(* Logix 5000 AddOnInstructionDefinition export GracoCore_DecodeDateTime; software revision 32.04; part 2 of 4 *)

ADD_ON_INSTRUCTION GracoPd2kDual_ReadJobInfo   (* revision 1.0 *)
// Help:
// Reads data from a job record.
// If indexNum is out of range, an error will be raised.
// State Codes:
// * 0000 (IDLE) - Idle
// * 1000 (BUSY) - Busy
// * 2000 (DONE) - Done
// * 4000 (ABORT) - Command overwritten by another process
// * 8000 (ERROR) - Index number out of range
// * 8001 (ERROR) - Timeout waiting for DCS registers
// * 8002 (ERROR) - Command unsuccessful
// * 8003 (ERROR) - Unhandled internal error
VAR_INPUT
   i_execute : BOOL; {visible}   // Execute command
   i_indexNum : DINT; {visible}   // Index number
END_VAR
VAR_IN_OUT
   io_userID : STRING9; {required}   // User ID
   io_moduleStatus : DINT[62]; {required}   // Data from device to PLC
   io_moduleCmds : DINT[30]; {required}   // Data from PLC to device
   io_dateTime : GracoCore_TypeDateTime; {required}   // Alarm/event datetime
END_VAR
VAR_OUTPUT
   o_mixUnitNum : DINT; {access Read Only, visible}   // Mix unit number
   o_jobNum : DINT; {access Read Only, visible}   // Job number
   o_recipeNum : DINT; {access Read Only, visible}   // Recipe number
   o_abVol : DINT; {access Read Only, visible}   // Material A+B used volume (cc)
   o_busy : BOOL; {access Read Only, visible}   // Busy flag
   o_done : BOOL; {access Read Only, visible}   // Done flag
   o_aborted : BOOL; {access Read Only, visible}   // Aborted flag
   o_error : BOOL; {access Read Only, visible}   // Error flag
   o_state : DINT; {access Read Only, visible}   // Command state
END_VAR
VAR
   sendDCSInst : GracoPd2kDual_SendDCS; {access None}   // SendDCS instruction
   decodeDateTime : GracoCore_DecodeDateTime; {access None}   // DecodeDateTime instruction
   decodeUserID : GracoCore_DecodeUserID; {access None}   // DecodeUserID instruction
END_VAR

ROUTINE Logic   (* ladder *)
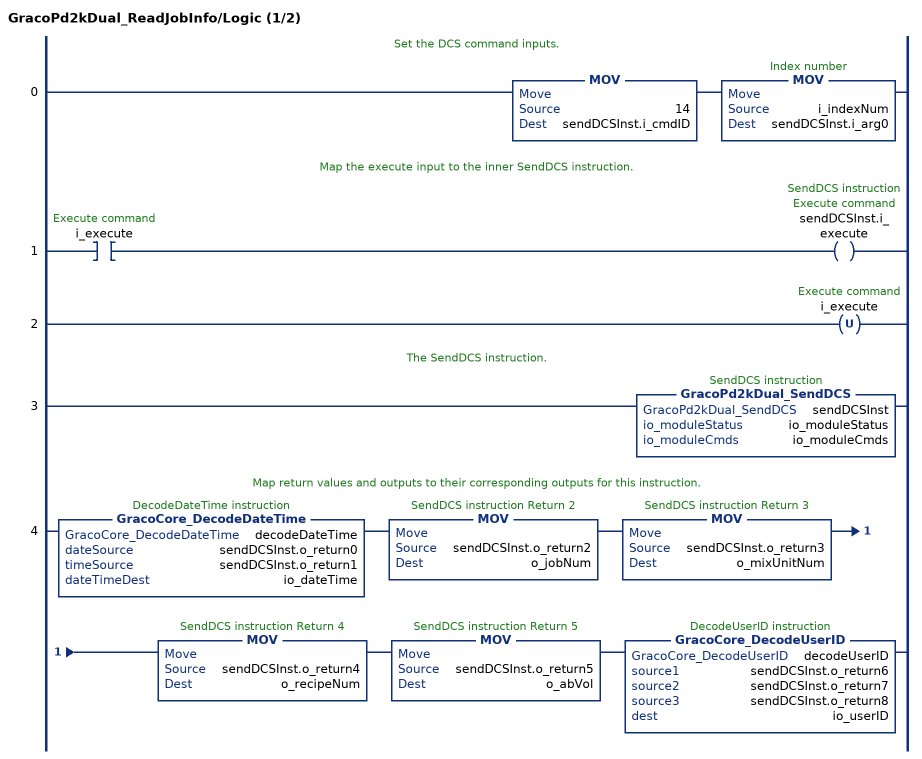
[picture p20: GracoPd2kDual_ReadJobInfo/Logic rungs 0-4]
   // Set the DCS command inputs.
   0: MOV(14,sendDCSInst.i_cmdID)MOV(i_indexNum,sendDCSInst.i_arg0);
   // Map the execute input to the inner SendDCS instruction.
   1: XIC(i_execute)OTE(sendDCSInst.i_execute);
   2: OTU(i_execute);
   // The SendDCS instruction.
   3: GracoPd2kDual_SendDCS(sendDCSInst,io_moduleStatus,io_moduleCmds);
   // Map return values and outputs to their corresponding outputs for this instruction.
   4: GracoCore_DecodeDateTime(decodeDateTime,sendDCSInst.o_return0,sendDCSInst.o_return1,io_dateTime)MOV(sendDCSInst.o_return2,o_jobNum)MOV(sendDCSInst.o_return3,o_mixUnitNum)MOV(sendDCSInst.o_return4,o_recipeNum)MOV(sendDCSInst.o_return5,o_abVol)GracoCore_DecodeUserID(decodeUserID,sendDCSInst.o_return6,sendDCSInst.o_return7,sendDCSInst.o_return8,io_userID);
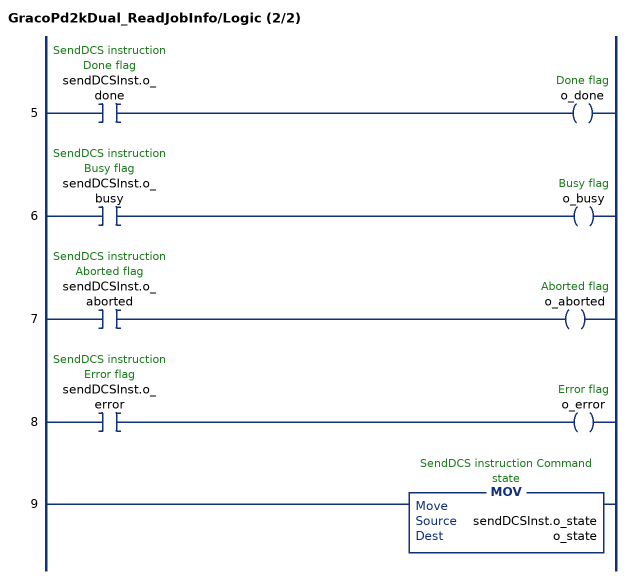
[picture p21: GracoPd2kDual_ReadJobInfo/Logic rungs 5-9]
   5: XIC(sendDCSInst.o_done)OTE(o_done);
   6: XIC(sendDCSInst.o_busy)OTE(o_busy);
   7: XIC(sendDCSInst.o_aborted)OTE(o_aborted);
   8: XIC(sendDCSInst.o_error)OTE(o_error);
   9: MOV(sendDCSInst.o_state,o_state);
END_ROUTINE
END_ADD_ON_INSTRUCTION

ADD_ON_INSTRUCTION GracoPd2kDual_ReadUserID   (* revision 1.0 *)
// Help:
// Returns the current user ID for the system.
// The returned value is a string of up to 9 characters, not including a null terminator.
// State Codes:
// * 0000 (IDLE) - Idle
// * 1000 (BUSY) - Busy
// * 2000 (DONE) - Done
// * 4000 (ABORT) - Command overwritten by another process
// * 8000 (ERROR) - Mix unit number out of range
// * 8001 (ERROR) - Timeout waiting for DCS registers
// * 8002 (ERROR) - Command unsuccessful
// * 8003 (ERROR) - Unhandled internal error
VAR_INPUT
   i_execute : BOOL; {visible}   // Execute command
   i_mixUnitNum : DINT; {visible}   // Mix unit number
END_VAR
VAR_IN_OUT
   io_userID : STRING9; {required}   // User ID
END_VAR
VAR_OUTPUT
   o_busy : BOOL; {access Read Only, visible}   // Busy flag
   o_done : BOOL; {access Read Only, visible}   // Done flag
   o_aborted : BOOL; {access Read Only, visible}   // Aborted flag
   o_error : BOOL; {access Read Only, visible}   // Error flag
   o_state : DINT; {access Read Only, visible}   // Command state
END_VAR
VAR_IN_OUT
   io_moduleStatus : DINT[62]; {required}   // Data from device to PLC
   io_moduleCmds : DINT[30]; {required}   // Data from PLC to device
END_VAR
VAR
   sendDCSInst : GracoPd2kDual_SendDCS; {access None}   // SendDCS instruction
   decodeUserID : GracoCore_DecodeUserID; {access None}   // DecodeUserID instruction
END_VAR

ROUTINE Logic   (* ladder *)
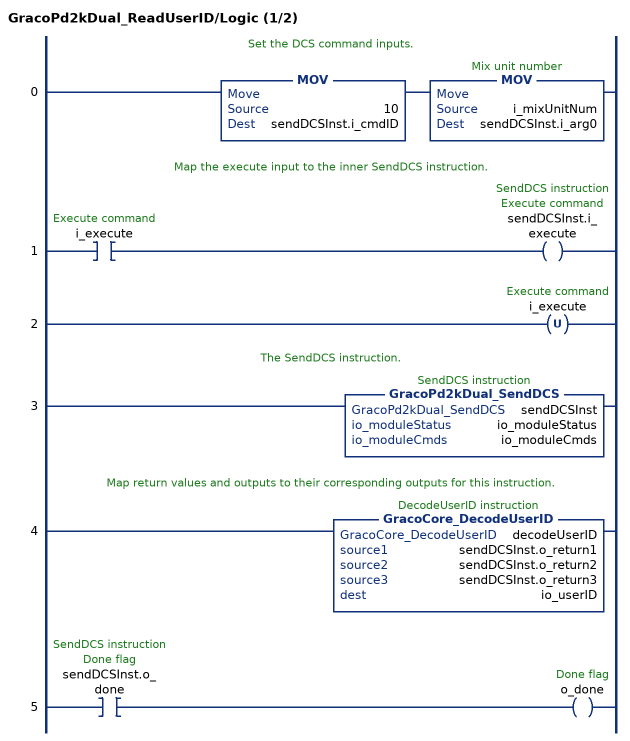
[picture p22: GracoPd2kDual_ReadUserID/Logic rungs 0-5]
   // Set the DCS command inputs.
   0: MOV(10,sendDCSInst.i_cmdID)MOV(i_mixUnitNum,sendDCSInst.i_arg0);
   // Map the execute input to the inner SendDCS instruction.
   1: XIC(i_execute)OTE(sendDCSInst.i_execute);
   2: OTU(i_execute);
   // The SendDCS instruction.
   3: GracoPd2kDual_SendDCS(sendDCSInst,io_moduleStatus,io_moduleCmds);
   // Map return values and outputs to their corresponding outputs for this instruction.
   4: GracoCore_DecodeUserID(decodeUserID,sendDCSInst.o_return1,sendDCSInst.o_return2,sendDCSInst.o_return3,io_userID);
   5: XIC(sendDCSInst.o_done)OTE(o_done);
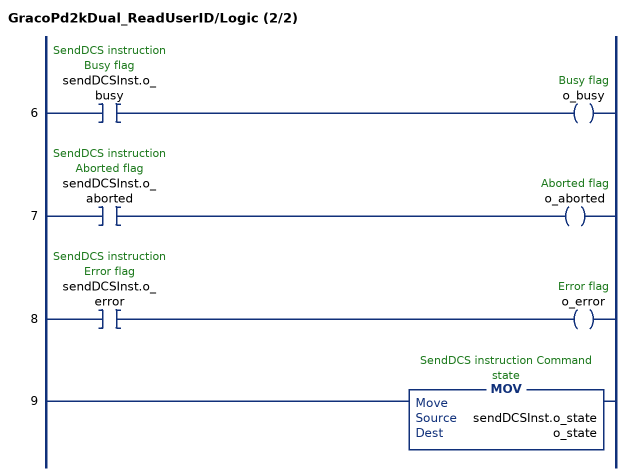
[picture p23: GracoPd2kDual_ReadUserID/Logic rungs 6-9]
   6: XIC(sendDCSInst.o_busy)OTE(o_busy);
   7: XIC(sendDCSInst.o_aborted)OTE(o_aborted);
   8: XIC(sendDCSInst.o_error)OTE(o_error);
   9: MOV(sendDCSInst.o_state,o_state);
END_ROUTINE
END_ADD_ON_INSTRUCTION

ADD_ON_INSTRUCTION GracoCore_EncodeUserID   (* revision 1.0 *)
// Help:
// Parses a user ID String (max 9 characters) into a series of ASCII values stored in DINTs. These can then be written to a Graco CGM.
VAR_IN_OUT
   source : STRING9; {required}
   dest1 : DINT; {required}
   dest2 : DINT; {required}
   dest3 : DINT; {required}
END_VAR
VAR
   buffer : DINT; {access None}
END_VAR

ROUTINE Logic   (* ladder *)
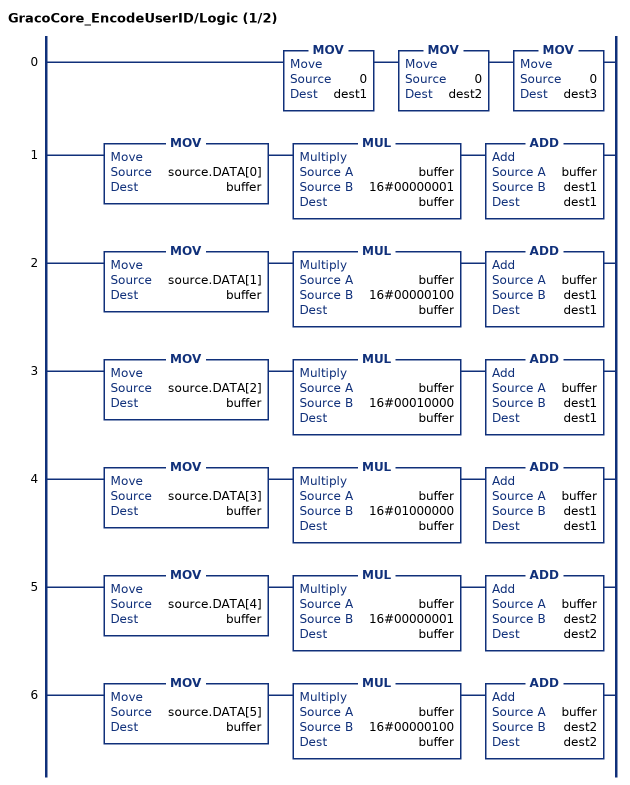
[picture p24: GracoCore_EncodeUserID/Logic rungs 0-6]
   0: MOV(0,dest1)MOV(0,dest2)MOV(0,dest3);
   1: MOV(source.DATA[0],buffer)MUL(buffer,16#00000001,buffer)ADD(buffer,dest1,dest1);
   2: MOV(source.DATA[1],buffer)MUL(buffer,16#00000100,buffer)ADD(buffer,dest1,dest1);
   3: MOV(source.DATA[2],buffer)MUL(buffer,16#00010000,buffer)ADD(buffer,dest1,dest1);
   4: MOV(source.DATA[3],buffer)MUL(buffer,16#01000000,buffer)ADD(buffer,dest1,dest1);
   5: MOV(source.DATA[4],buffer)MUL(buffer,16#00000001,buffer)ADD(buffer,dest2,dest2);
   6: MOV(source.DATA[5],buffer)MUL(buffer,16#00000100,buffer)ADD(buffer,dest2,dest2);
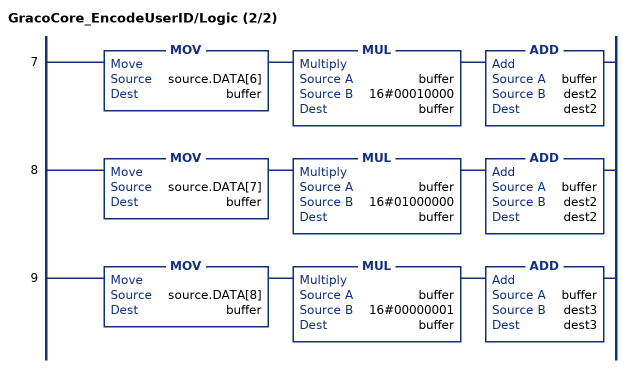
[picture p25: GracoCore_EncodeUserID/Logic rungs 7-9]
   7: MOV(source.DATA[6],buffer)MUL(buffer,16#00010000,buffer)ADD(buffer,dest2,dest2);
   8: MOV(source.DATA[7],buffer)MUL(buffer,16#01000000,buffer)ADD(buffer,dest2,dest2);
   9: MOV(source.DATA[8],buffer)MUL(buffer,16#00000001,buffer)ADD(buffer,dest3,dest3);
END_ROUTINE
END_ADD_ON_INSTRUCTION

ADD_ON_INSTRUCTION GracoPd2kDual_WriteUserID   (* revision 1.0 *)
// Help:
// Sets the current user ID for the system.
// The user ID can be up to 9 characters in length. The value sent to the PD2K will include a null terminator for a total of 10 characters. Only ASCII characters are supported.
// State Codes:
// * 0000 (IDLE) - Idle
// * 1000 (BUSY) - Busy
// * 2000 (DONE) - Done
// * 4000 (ABORT) - Command overwritten by another process
// * 8000 (ERROR) - Mix unit number out of range
// * 8001 (ERROR) - Timeout waiting for DCS registers
// * 8002 (ERROR) - Command unsuccessful
// * 8003 (ERROR) - Unhandled internal error
VAR_INPUT
   i_execute : BOOL; {visible}   // Execute command
END_VAR
VAR_IN_OUT
   io_userID : STRING9; {required}   // User ID
END_VAR
VAR_OUTPUT
   o_busy : BOOL; {access Read Only, visible}   // Busy flag
   o_done : BOOL; {access Read Only, visible}   // Done flag
   o_aborted : BOOL; {access Read Only, visible}   // Aborted flag
   o_error : BOOL; {access Read Only, visible}   // Error flag
   o_state : DINT; {access Read Only, visible}   // Command state
END_VAR
VAR_IN_OUT
   io_moduleStatus : DINT[62]; {required}   // Data from device to PLC
   io_moduleCmds : DINT[30]; {required}   // Data from PLC to device
END_VAR
VAR_INPUT
   i_mixUnitNum : DINT; {visible}   // Mix unit number
END_VAR
VAR
   sendDCSInst : GracoPd2kDual_SendDCS; {access None}   // SendDCS instruction
   encodeUserID : GracoCore_EncodeUserID; {access None}   // EncodeUserID instruction
END_VAR

ROUTINE Logic   (* ladder *)
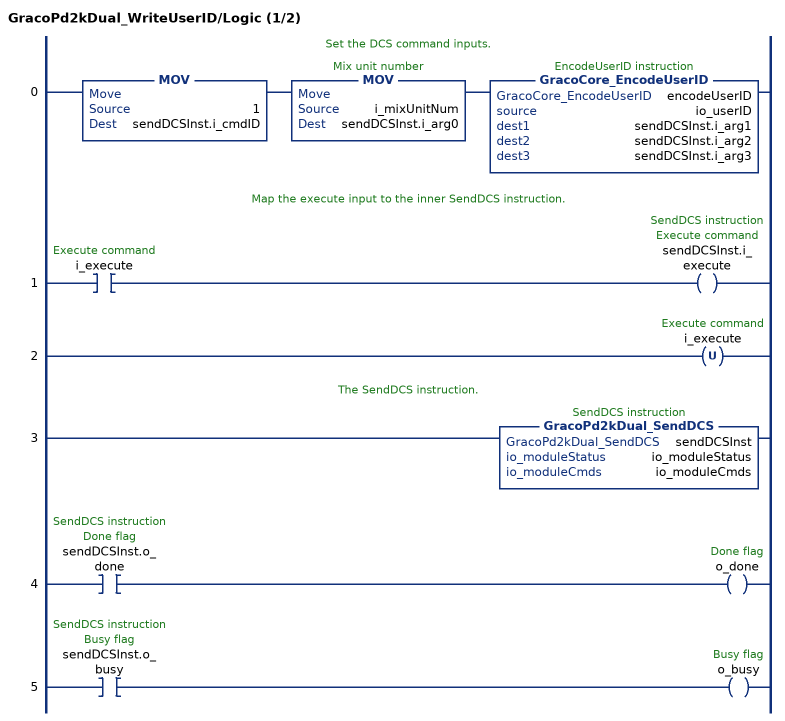
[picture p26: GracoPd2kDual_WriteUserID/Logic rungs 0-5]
   // Set the DCS command inputs.
   0: MOV(1,sendDCSInst.i_cmdID)MOV(i_mixUnitNum,sendDCSInst.i_arg0)GracoCore_EncodeUserID(encodeUserID,io_userID,sendDCSInst.i_arg1,sendDCSInst.i_arg2,sendDCSInst.i_arg3);
   // Map the execute input to the inner SendDCS instruction.
   1: XIC(i_execute)OTE(sendDCSInst.i_execute);
   2: OTU(i_execute);
   // The SendDCS instruction.
   3: GracoPd2kDual_SendDCS(sendDCSInst,io_moduleStatus,io_moduleCmds);
   4: XIC(sendDCSInst.o_done)OTE(o_done);
   5: XIC(sendDCSInst.o_busy)OTE(o_busy);
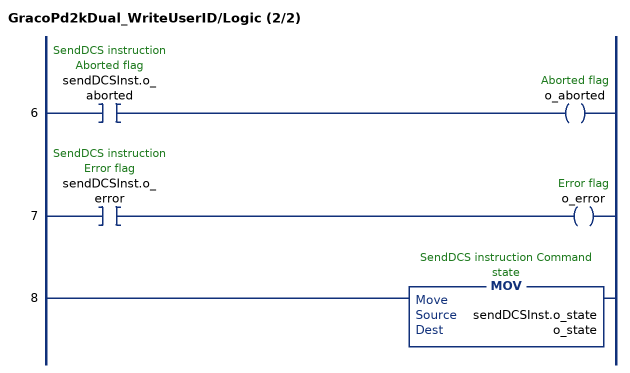
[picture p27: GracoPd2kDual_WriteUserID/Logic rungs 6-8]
   6: XIC(sendDCSInst.o_aborted)OTE(o_aborted);
   7: XIC(sendDCSInst.o_error)OTE(o_error);
   8: MOV(sendDCSInst.o_state,o_state);
END_ROUTINE
END_ADD_ON_INSTRUCTION

ADD_ON_INSTRUCTION GracoCore_Step   (* revision 1.0 *)
// Help:
// An implementation of the step pattern, useful for sequences in ladder logic.
VAR_INPUT
   doneTrigger : BOOL; {access None, visible}
   preCond : BOOL; {visible}
END_VAR
VAR_OUTPUT
   isDone : BOOL; {access Read Only, visible}
   isRunning : BOOL; {access None, visible}
END_VAR

ROUTINE Logic   (* ladder *)
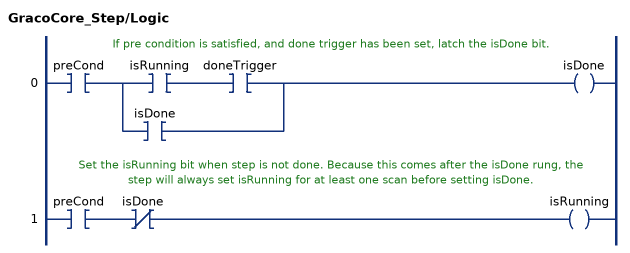
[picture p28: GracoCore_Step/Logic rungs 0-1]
   // If pre condition is satisfied, and done trigger has been set, latch the isDone bit.
   0: XIC(preCond)[XIC(isRunning) XIC(doneTrigger) ,XIC(isDone) ]OTE(isDone);
   // Set the isRunning bit when step is not done. Because this comes after the isDone rung, the step will always set isRunning for at least one scan before setting isDone.
   1: XIC(preCond)XIO(isDone)OTE(isRunning);
END_ROUTINE
END_ADD_ON_INSTRUCTION

ADD_ON_INSTRUCTION GracoPd2kDual_MainCtrl   (* revision 1.0 *)
// Help:
// Provides several inputs for controlling the PD2K proportioner (e.g. system mode, setpoints).
// The enable input must be on for any other inputs to take effect. The boolean command inputs each function like execute inputs, meaning the command will automatically reset these once set to true.
// The current control mode setting (pressure or flow) determines which of the setpoint inputs are written to the PD2K system. This switches automatically when the control mode is changed.
// State Codes:
// * 0000 (IDLE) - Idle
// * 3000 (VALID) - Valid
// * 8000 (ERROR) - Invalid mix unit number
VAR_INPUT
   i_clearAlarm : BOOL; {visible}   // Clear alarm
   i_completeJob : BOOL; {visible}   // Complete job
   i_ctrlMode : BOOL; {visible}   // Ctrl mode SP (0=flow, 1=pressure)
   i_enable : BOOL; {visible}   // Enable command
   i_mix : BOOL; {visible}   // Goto mix
   i_mixFill : BOOL; {visible}   // Goto mix fill
   i_powerOff : BOOL; {visible}   // Power off
   i_powerOn : BOOL; {visible}   // Power on
   i_quickStop : BOOL; {visible}   // Goto quick stop
   i_recipePurge : BOOL; {visible}   // Goto recipe purge
   i_standby : BOOL; {visible}   // Goto standby
   i_mixUnitNum : DINT; {visible}   // Mix unit number (1-2)
   i_flowCtrlSP : DINT; {visible}   // Flow control setpoint (cc/min)
   i_presCtrlSP : DINT; {visible}   // Pressure control setpoint (psi)
END_VAR
VAR_IN_OUT
   io_moduleStatus : DINT[62]; {required}   // Data from module to PLC
   io_moduleCmds : DINT[30]; {required}   // Data from PLC to module
END_VAR
VAR_OUTPUT
   o_aborted : BOOL; {access Read Only, visible}   // Command aborted flag
   o_busy : BOOL; {access Read Only, visible}   // Busy flag
   o_error : BOOL; {access Read Only, visible}   // Error flag
   o_valid : BOOL; {access Read Only, visible}   // Command valid flag
   o_state : DINT; {access Read Only, visible}   // Command state
END_VAR
VAR
   clearAlmPBTmr : TIMER := (PRE := 250); {access None}   // Clear alarm pushbutton timer
   jobCompletePBTmr : TIMER := (PRE := 250); {access None}   // Job complete input timer
   mixFillPBTmr : TIMER := (PRE := 250); {access None}   // Mix fill input timer
   mixPBTmr : TIMER := (PRE := 250); {access None}   // Mix input timer
   ons : DINT; {access None}   // oneshot
   powerOnPBTmr : TIMER := (PRE := 250); {access None}   // Power on input timer
   pumpIsOff : BOOL; {access None}   // Pump is off
   purgePBTmr : TIMER := (PRE := 250); {access None}   // Purge input timer
   quickStopPBTmr : TIMER := (PRE := 250); {access None}   // Quick stop input timer
   isStandby : BOOL; {access None}   // System is in standby
   toStandbyPBTmr : TIMER := (PRE := 250); {access None}   // Standby input timer
   _mixUnitNum : DINT; {access None}   // Mix unit number (internal)
   mixUnitNumOK : BOOL; {access None}   // Mix unit number OK
   systemCmdAvailable : BOOL; {access None}   // System command register is available
   powerOnOffSetTrigger : BOOL; {access None}   // Power on/off set trigger
   powerOnOffResetTrigger : BOOL; {access None}   // Power on/off reset trigger
   quickStopSetTrigger : BOOL; {access None}   // Quick stop set trigger
   quickStopResetTrigger : BOOL; {access None}   // Quick stop reset trigger
   mixFillSetTrigger : BOOL; {access None}   // Mix fill set trigger
   mixFillResetTrigger : BOOL; {access None}   // Mix fill reset trigger
   mixSetTrigger : BOOL; {access None}   // Mix set trigger
   mixResetTrigger : BOOL; {access None}   // Mix reset trigger
   toStandbySetTrigger : BOOL; {access None}   // Standby set trigger
   toStandbyResetTrigger : BOOL; {access None}   // Standby reset trigger
   purgeSetTrigger : BOOL; {access None}   // Purge set trigger
   purgeResetTrigger : BOOL; {access None}   // Purge reset trigger
   state_idle : DINT; {access None}
   state_checkInputs : DINT; {access None}
   state_update : DINT; {access None}
   _nextState : DINT; {access None}
   state_errorInvalidMixUnitNum : DINT; {access None}
END_VAR

ROUTINE Logic   (* ladder *)
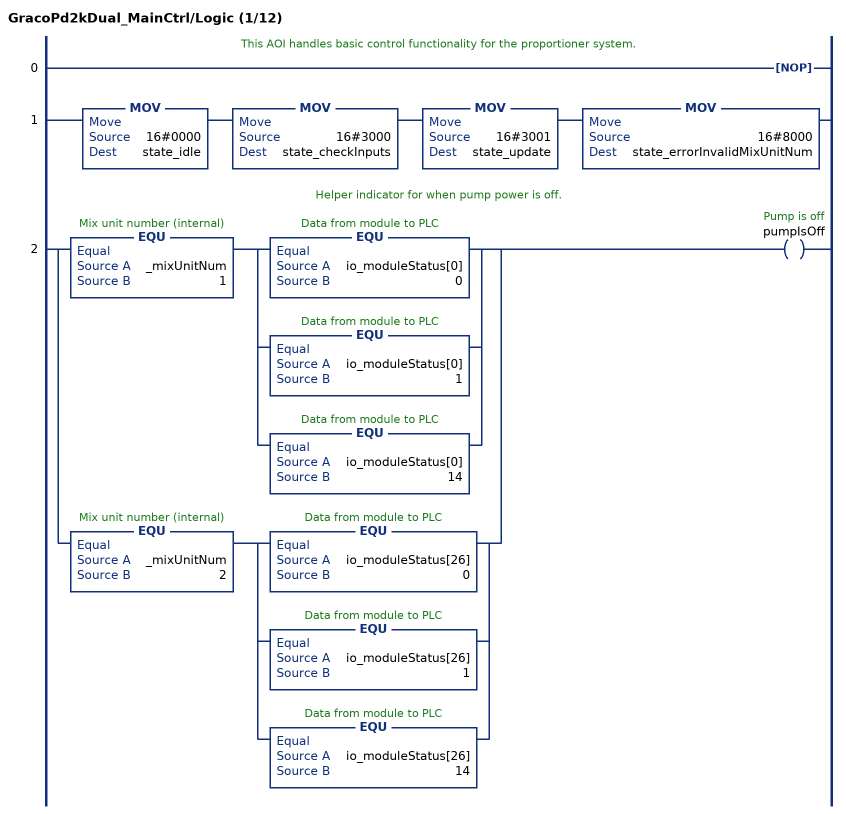
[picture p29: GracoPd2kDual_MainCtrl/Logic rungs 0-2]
   // This AOI handles basic control functionality for the proportioner system.
   0: NOP();
   1: MOV(16#0000,state_idle)MOV(16#3000,state_checkInputs)MOV(16#3001,state_update)MOV(16#8000,state_errorInvalidMixUnitNum);
   // Helper indicator for when pump power is off.
   2: [EQU(_mixUnitNum,1) [EQU(io_moduleStatus[0],0) ,EQU(io_moduleStatus[0],1) ,EQU(io_moduleStatus[0],14) ] ,EQU(_mixUnitNum,2) [EQU(io_moduleStatus[26],0) ,EQU(io_moduleStatus[26],1) ,EQU(io_moduleStatus[26],14) ] ]OTE(pumpIsOff);
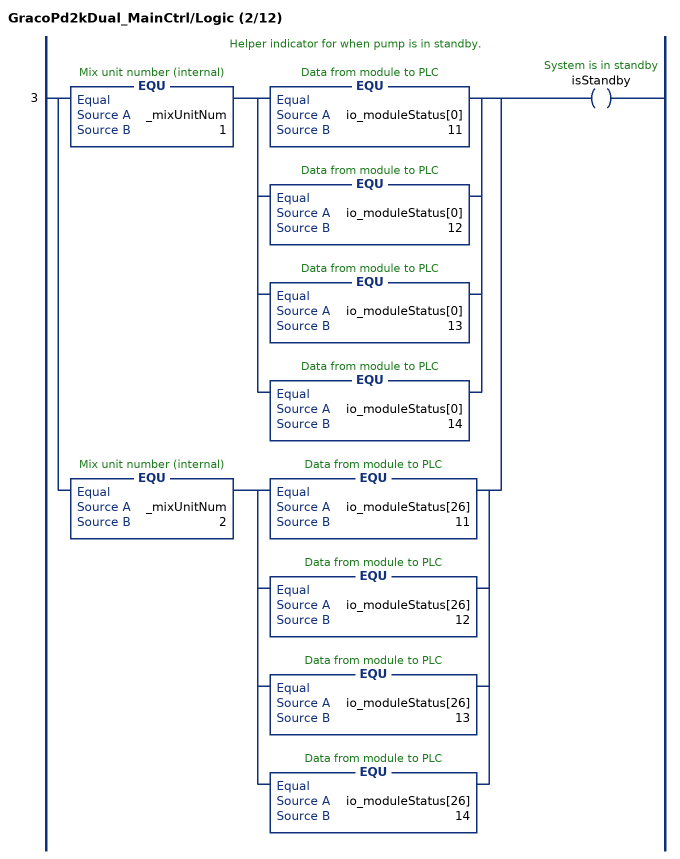
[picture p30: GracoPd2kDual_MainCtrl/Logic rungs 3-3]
   // Helper indicator for when pump is in standby.
   3: [EQU(_mixUnitNum,1) [EQU(io_moduleStatus[0],11) ,EQU(io_moduleStatus[0],12) ,EQU(io_moduleStatus[0],13) ,EQU(io_moduleStatus[0],14) ] ,EQU(_mixUnitNum,2) [EQU(io_moduleStatus[26],11) ,EQU(io_moduleStatus[26],12) ,EQU(io_moduleStatus[26],13) ,EQU(io_moduleStatus[26],14) ] ]OTE(isStandby);
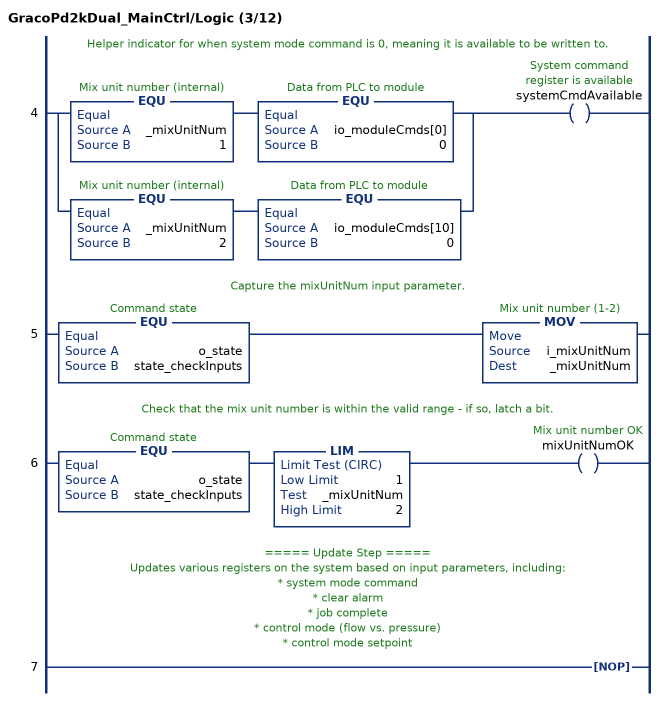
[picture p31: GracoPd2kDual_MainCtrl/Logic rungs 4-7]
   // Helper indicator for when system mode command is 0, meaning it is available to be written to.
   4: [EQU(_mixUnitNum,1) EQU(io_moduleCmds[0],0) ,EQU(_mixUnitNum,2) EQU(io_moduleCmds[10],0) ]OTE(systemCmdAvailable);
   // Capture the mixUnitNum input parameter.
   5: EQU(o_state,state_checkInputs)MOV(i_mixUnitNum,_mixUnitNum);
   // Check that the mix unit number is within the valid range - if so, latch a bit.
   6: EQU(o_state,state_checkInputs)LIM(1,_mixUnitNum,2)OTE(mixUnitNumOK);
   // ===== Update Step =====
   // Updates various registers on the system based on input parameters, including:
   // * system mode command
   // * clear alarm
   // * job complete
   // * control mode (flow vs. pressure)
   // * control mode setpoint
   7: NOP();
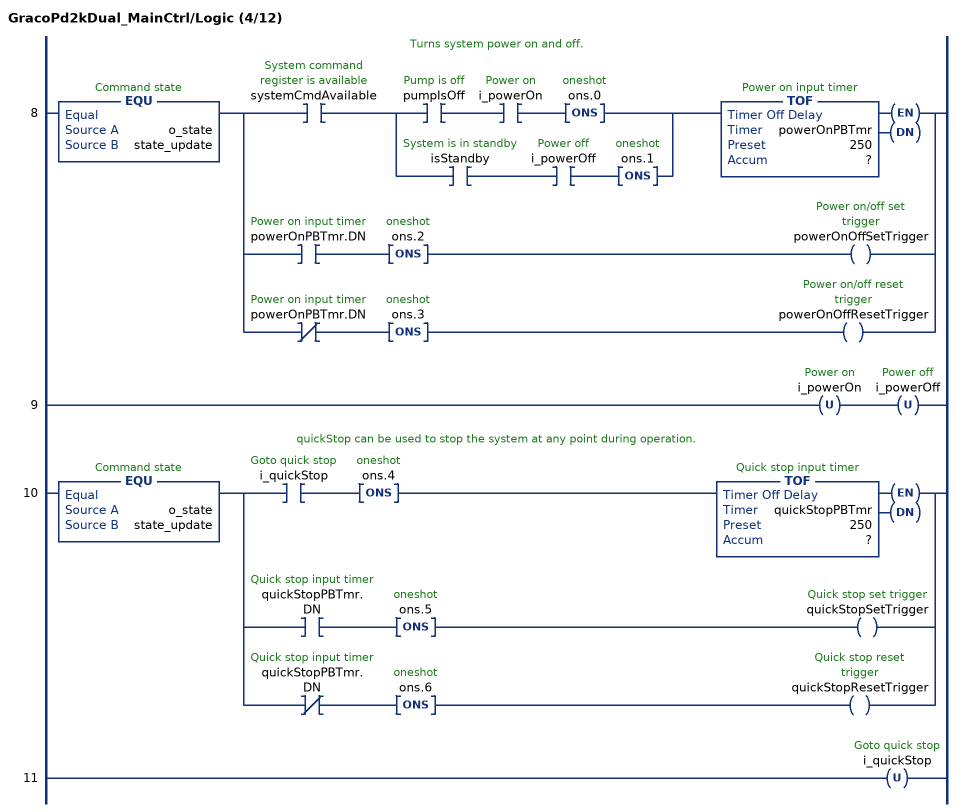
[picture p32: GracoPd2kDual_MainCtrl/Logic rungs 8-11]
   // Turns system power on and off.
   8: EQU(o_state,state_update)[XIC(systemCmdAvailable) [XIC(pumpIsOff) XIC(i_powerOn) ONS(ons.0) ,XIC(isStandby) XIC(i_powerOff) ONS(ons.1) ] TOF(powerOnPBTmr,?,?) ,XIC(powerOnPBTmr.DN) ONS(ons.2) OTE(powerOnOffSetTrigger) ,XIO(powerOnPBTmr.DN) ONS(ons.3) OTE(powerOnOffResetTrigger) ];
   9: OTU(i_powerOn)OTU(i_powerOff);
   // quickStop can be used to stop the system at any point during operation.
   10: EQU(o_state,state_update)[XIC(i_quickStop) ONS(ons.4) TOF(quickStopPBTmr,?,?) ,XIC(quickStopPBTmr.DN) ONS(ons.5) OTE(quickStopSetTrigger) ,XIO(quickStopPBTmr.DN) ONS(ons.6) OTE(quickStopResetTrigger) ];
   11: OTU(i_quickStop);
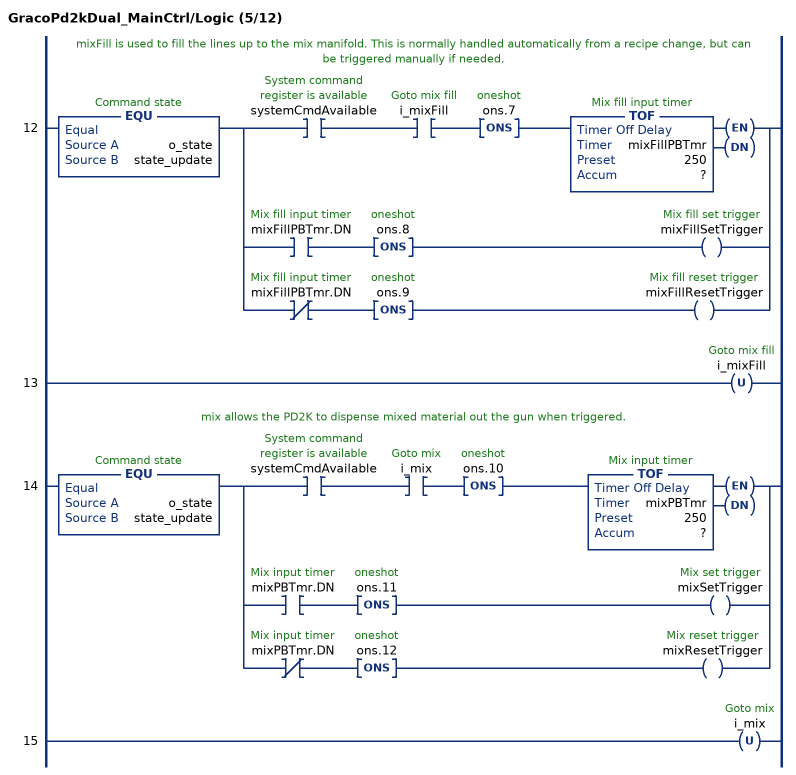
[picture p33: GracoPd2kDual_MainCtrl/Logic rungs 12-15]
   // mixFill is used to fill the lines up to the mix manifold. This is normally handled automatically from a recipe change, but can be triggered manually if needed.
   12: EQU(o_state,state_update)[XIC(systemCmdAvailable) XIC(i_mixFill) ONS(ons.7) TOF(mixFillPBTmr,?,?) ,XIC(mixFillPBTmr.DN) ONS(ons.8) OTE(mixFillSetTrigger) ,XIO(mixFillPBTmr.DN) ONS(ons.9) OTE(mixFillResetTrigger) ];
   13: OTU(i_mixFill);
   // mix allows the PD2K to dispense mixed material out the gun when triggered.
   14: EQU(o_state,state_update)[XIC(systemCmdAvailable) XIC(i_mix) ONS(ons.10) TOF(mixPBTmr,?,?) ,XIC(mixPBTmr.DN) ONS(ons.11) OTE(mixSetTrigger) ,XIO(mixPBTmr.DN) ONS(ons.12) OTE(mixResetTrigger) ];
   15: OTU(i_mix);
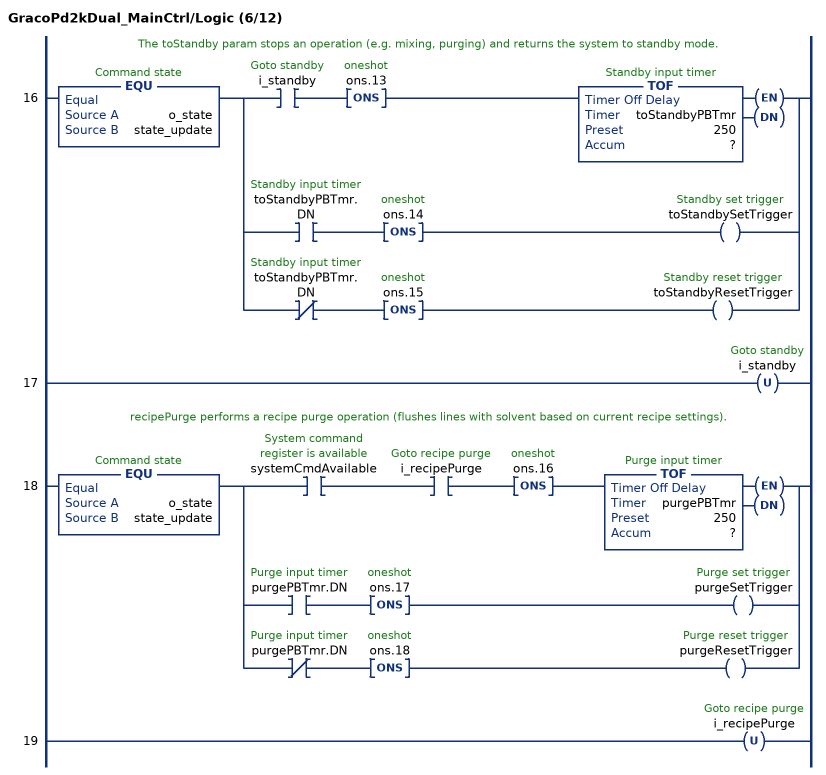
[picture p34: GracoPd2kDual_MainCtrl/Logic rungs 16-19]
   // The toStandby param stops an operation (e.g. mixing, purging) and returns the system to standby mode.
   16: EQU(o_state,state_update)[XIC(i_standby) ONS(ons.13) TOF(toStandbyPBTmr,?,?) ,XIC(toStandbyPBTmr.DN) ONS(ons.14) OTE(toStandbySetTrigger) ,XIO(toStandbyPBTmr.DN) ONS(ons.15) OTE(toStandbyResetTrigger) ];
   17: OTU(i_standby);
   // recipePurge performs a recipe purge operation (flushes lines with solvent based on current recipe settings).
   18: EQU(o_state,state_update)[XIC(systemCmdAvailable) XIC(i_recipePurge) ONS(ons.16) TOF(purgePBTmr,?,?) ,XIC(purgePBTmr.DN) ONS(ons.17) OTE(purgeSetTrigger) ,XIO(purgePBTmr.DN) ONS(ons.18) OTE(purgeResetTrigger) ];
   19: OTU(i_recipePurge);
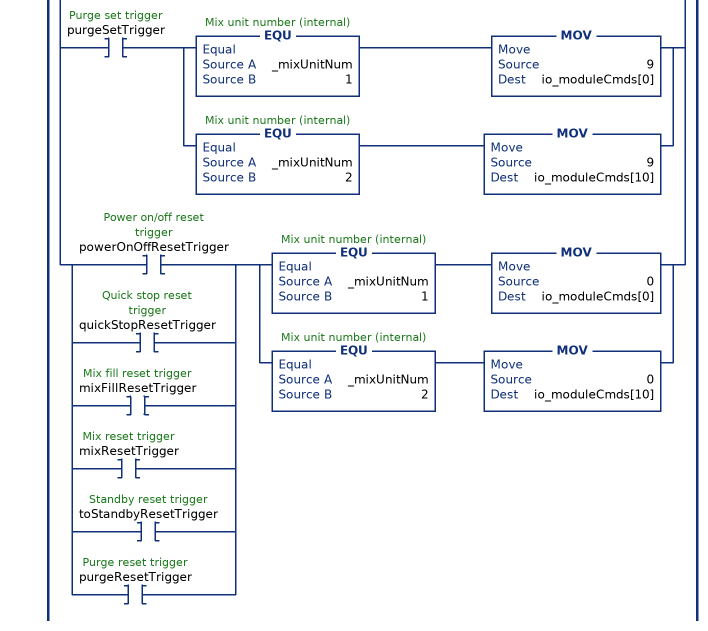
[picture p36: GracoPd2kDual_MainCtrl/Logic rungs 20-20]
   // Write the system mode command register depending on the mix unit number and any triggers driven from the input parameters.
   20: [XIC(powerOnOffSetTrigger) [EQU(_mixUnitNum,1) MOV(1,io_moduleCmds[0]) ,EQU(_mixUnitNum,2) MOV(1,io_moduleCmds[10]) ] ,XIC(quickStopSetTrigger) [EQU(_mixUnitNum,1) MOV(2,io_moduleCmds[0]) ,EQU(_mixUnitNum,2) MOV(2,io_moduleCmds[10]) ] ,XIC(mixFillSetTrigger) [EQU(_mixUnitNum,1) MOV(4,io_moduleCmds[0]) ,EQU(_mixUnitNum,2) MOV(4,io_moduleCmds[10]) ] ,XIC(mixSetTrigger) [EQU(_mixUnitNum,1) MOV(5,io_moduleCmds[0]) ,EQU(_mixUnitNum,2) MOV(5,io_moduleCmds[10]) ] ,XIC(toStandbySetTrigger) [EQU(_mixUnitNum,1) MOV(8,io_moduleCmds[0]) ,EQU(_mixUnitNum,2) MOV(8,io_moduleCmds[10]) ] ,XIC(purgeSetTrigger) [EQU(_mixUnitNum,1) MOV(9,io_moduleCmds[0]) ,EQU(_mixUnitNum,2) MOV(9,io_moduleCmds[10]) ] ,[XIC(powerOnOffResetTrigger) ,XIC(quickStopResetTrigger) ,XIC(mixFillResetTrigger) ,XIC(mixResetTrigger) ,XIC(toStandbyResetTrigger) ,XIC(purgeResetTrigger) ] [EQU(_mixUnitNum,1) MOV(0,io_moduleCmds[0]) ,EQU(_mixUnitNum,2) MOV(0,io_moduleCmds[10]) ] ];
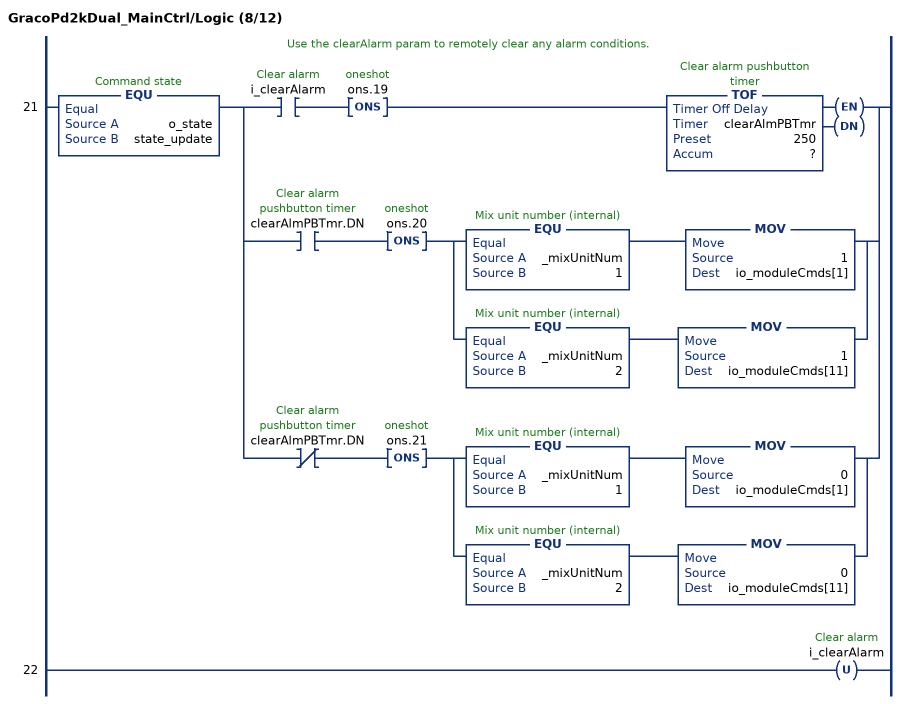
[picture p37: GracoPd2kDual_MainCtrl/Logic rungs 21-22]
   // Use the clearAlarm param to remotely clear any alarm conditions.
   21: EQU(o_state,state_update)[XIC(i_clearAlarm) ONS(ons.19) TOF(clearAlmPBTmr,?,?) ,XIC(clearAlmPBTmr.DN) ONS(ons.20) [EQU(_mixUnitNum,1) MOV(1,io_moduleCmds[1]) ,EQU(_mixUnitNum,2) MOV(1,io_moduleCmds[11]) ] ,XIO(clearAlmPBTmr.DN) ONS(ons.21) [EQU(_mixUnitNum,1) MOV(0,io_moduleCmds[1]) ,EQU(_mixUnitNum,2) MOV(0,io_moduleCmds[11]) ] ];
   22: OTU(i_clearAlarm);
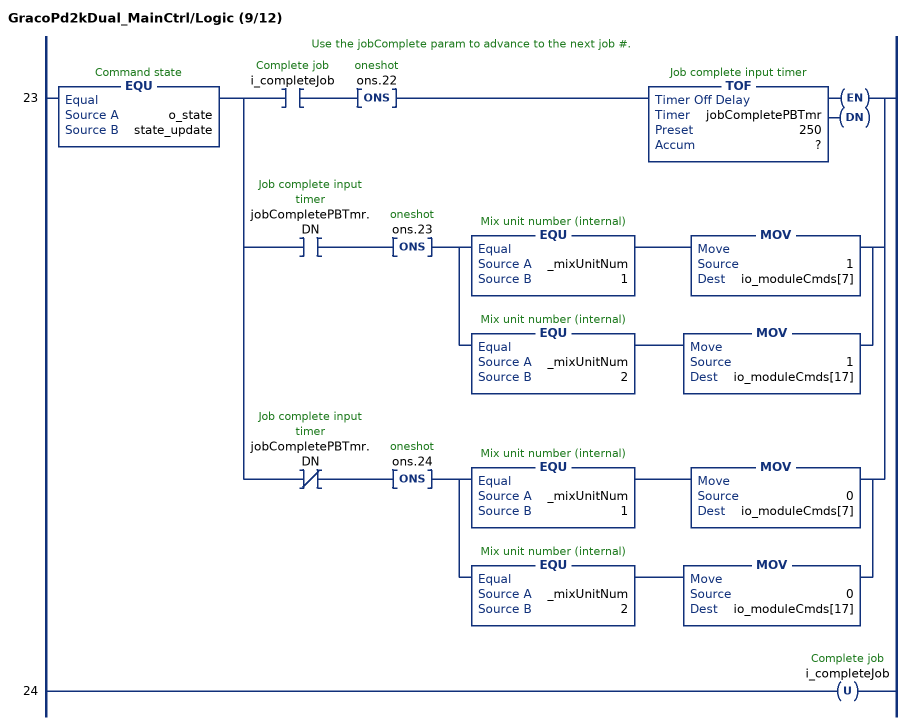
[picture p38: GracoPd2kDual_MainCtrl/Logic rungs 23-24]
   // Use the jobComplete param to advance to the next job #.
   23: EQU(o_state,state_update)[XIC(i_completeJob) ONS(ons.22) TOF(jobCompletePBTmr,?,?) ,XIC(jobCompletePBTmr.DN) ONS(ons.23) [EQU(_mixUnitNum,1) MOV(1,io_moduleCmds[7]) ,EQU(_mixUnitNum,2) MOV(1,io_moduleCmds[17]) ] ,XIO(jobCompletePBTmr.DN) ONS(ons.24) [EQU(_mixUnitNum,1) MOV(0,io_moduleCmds[7]) ,EQU(_mixUnitNum,2) MOV(0,io_moduleCmds[17]) ] ];
   24: OTU(i_completeJob);
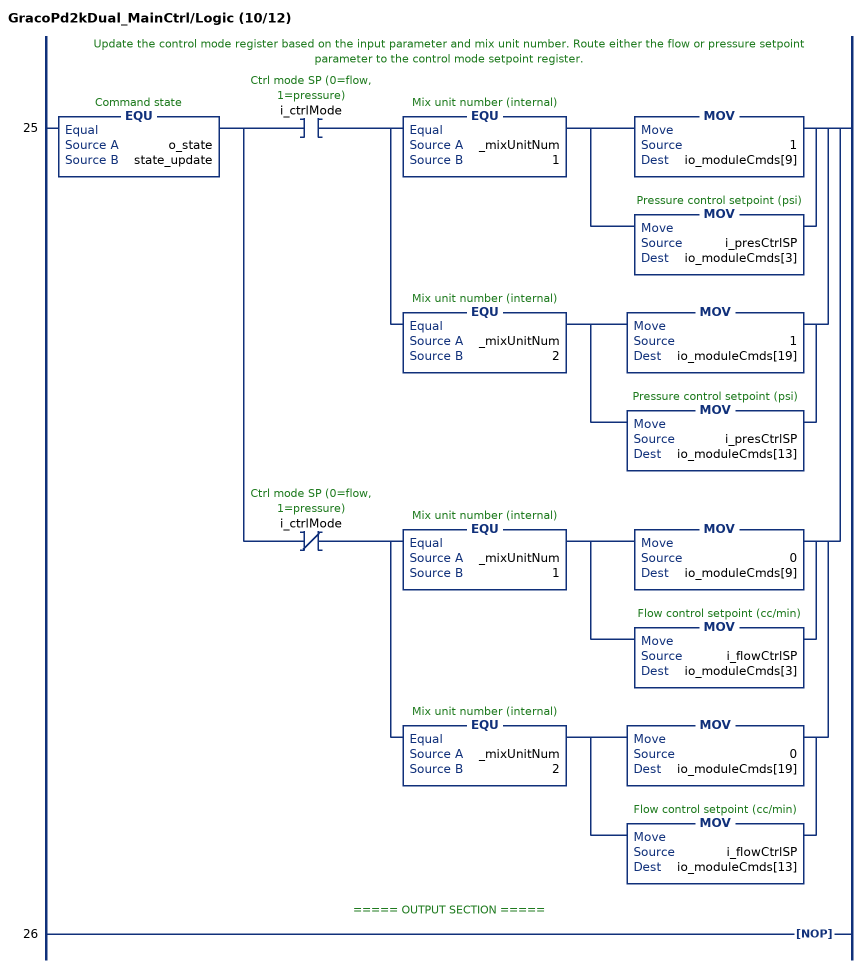
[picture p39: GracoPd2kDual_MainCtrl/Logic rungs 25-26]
   // Update the control mode register based on the input parameter and mix unit number. Route either the flow or pressure setpoint parameter to the control mode setpoint register.
   25: EQU(o_state,state_update)[XIC(i_ctrlMode) [EQU(_mixUnitNum,1) [MOV(1,io_moduleCmds[9]) ,MOV(i_presCtrlSP,io_moduleCmds[3]) ] ,EQU(_mixUnitNum,2) [MOV(1,io_moduleCmds[19]) ,MOV(i_presCtrlSP,io_moduleCmds[13]) ] ] ,XIO(i_ctrlMode) [EQU(_mixUnitNum,1) [MOV(0,io_moduleCmds[9]) ,MOV(i_flowCtrlSP,io_moduleCmds[3]) ] ,EQU(_mixUnitNum,2) [MOV(0,io_moduleCmds[19]) ,MOV(i_flowCtrlSP,io_moduleCmds[13]) ] ] ];
   // ===== OUTPUT SECTION =====
   26: NOP();
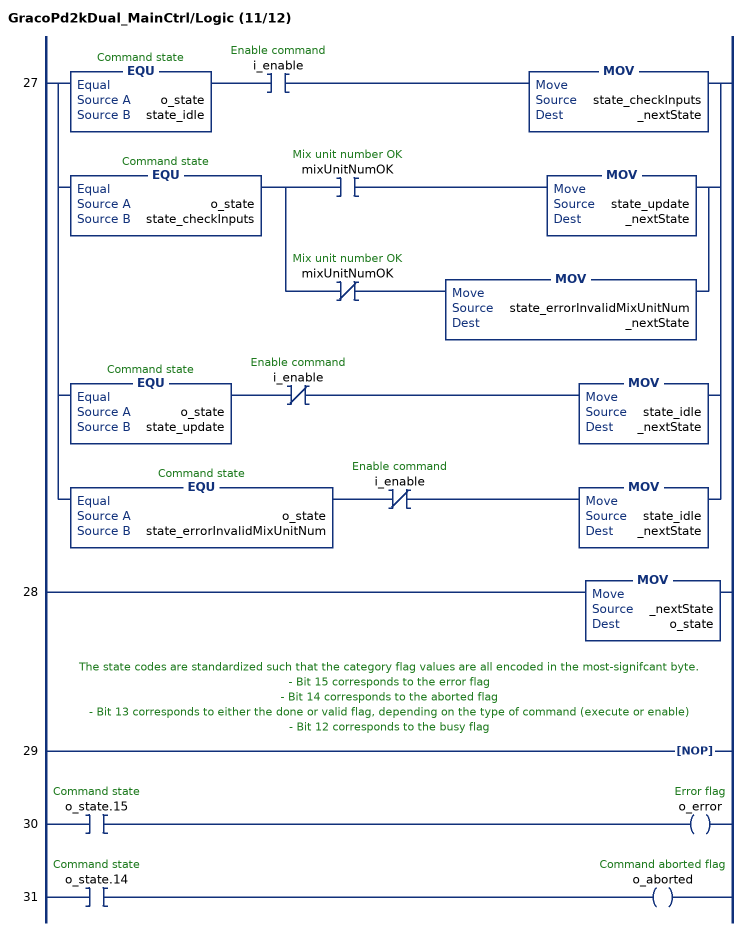
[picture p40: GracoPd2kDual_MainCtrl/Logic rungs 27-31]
   27: [EQU(o_state,state_idle) XIC(i_enable) MOV(state_checkInputs,_nextState) ,EQU(o_state,state_checkInputs) [XIC(mixUnitNumOK) MOV(state_update,_nextState) ,XIO(mixUnitNumOK) MOV(state_errorInvalidMixUnitNum,_nextState) ] ,EQU(o_state,state_update) XIO(i_enable) MOV(state_idle,_nextState) ,EQU(o_state,state_errorInvalidMixUnitNum) XIO(i_enable) MOV(state_idle,_nextState) ];
   28: MOV(_nextState,o_state);
   // The state codes are standardized such that the category flag values are all encoded in the most-signifcant byte.
   // - Bit 15 corresponds to the error flag
   // - Bit 14 corresponds to the aborted flag
   // - Bit 13 corresponds to either the done or valid flag, depending on the type of command (execute or enable)
   // - Bit 12 corresponds to the busy flag
   29: NOP();
   30: XIC(o_state.15)OTE(o_error);
   31: XIC(o_state.14)OTE(o_aborted);
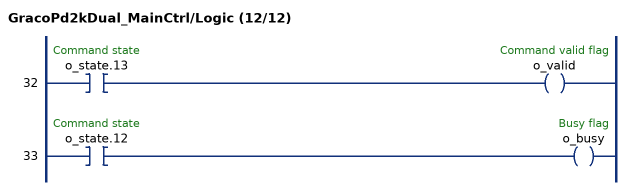
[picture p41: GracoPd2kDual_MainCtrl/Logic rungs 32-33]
   32: XIC(o_state.13)OTE(o_valid);
   33: XIC(o_state.12)OTE(o_busy);
END_ROUTINE
END_ADD_ON_INSTRUCTION
